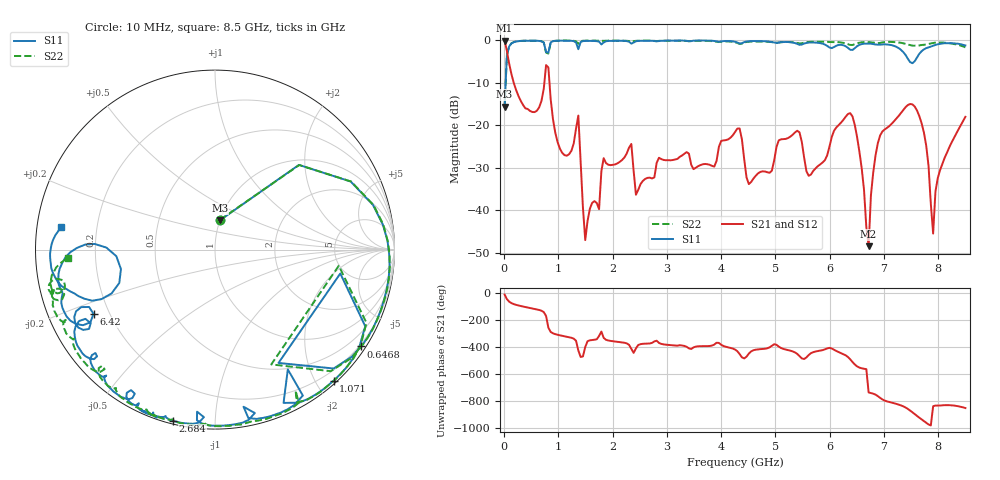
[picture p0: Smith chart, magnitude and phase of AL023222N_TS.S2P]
!AVX CORPORATION
!PN: AL023222N_TS
!DESCRIPTION: AIR CORE INDUCTOR, 222nH, 14 turns
!Agilent Technologies,E5071C,MY46102230,A.09.54
!Date: Mon Sep 03 16:46:35 2012
!Data & Calibration Information:
!Freq	S11:SOLT2(ON)	S21:SOLT2(ON)	S12:SOLT2(ON)	S22:SOLT2(ON)
# Hz S dB R 50
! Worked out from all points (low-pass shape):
!   201 points, 10 MHz to 8.5 GHz, reference 50 ohm
!   highest |S21| = -0.11 dB at 10 MHz (marker M1); lowest = -48.4 dB at 6.717 GHz (marker M2)
!   |S21| within 3 dB of the highest: start of sweep to 60.05 MHz
!   lowest |S11| = -15.6 dB at 10 MHz (marker M3), VSWR 1.40, Z = 50 + j16.8 ohm
!   |S11| at or under -10 dB: start of sweep to 29.75 MHz
!   |S22| runs from -15.5 to -0.1 dB; largest |S21 - S12| = 0.0023
!   S11 on the Smith chart (normalised r, x): 10 MHz: 1.00, +0.34; 646.8 MHz: 0.14, -3.32; 1.071 GHz: 0.05, -2.25; 2.684 GHz: 0.01, -0.78; 6.42 GHz: 0.14, -0.24; 8.5 GHz: 0.07, +0.07
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1e7  -15.61 80.4  -0.11 -10.2  -0.10 -10.2  -15.54 80.9
1.798e8  -0.49 8.5  -10.10 -81.1  -10.08 -81.1  -0.46 8.4
6.4675e8  -0.20 -33.5  -15.80 -124.4  -15.80 -124.4  -0.19 -34.1
8.1655e8  -2.97 -10.8  -6.44 103.8  -6.43 103.8  -3.15 -7.4
1.07125e9  -0.13 -47.8  -26.49 44.3  -26.48 44.2  -0.12 -47.1
1.3684e9  -2.14 -58.7  -17.74 -64.2  -17.73 -64.1  -0.87 -60.2
1.4533e9  -0.25 -62.9  -39.40 -108.3  -39.58 -108.7  -0.16 -63.9
2.34475e9  -0.83 -96.3  -24.40 -51.7  -24.40 -51.6  -0.35 -93.8
2.42965e9  -0.28 -95.4  -36.32 -48.9  -36.45 -49.9  -0.17 -95.0
2.68435e9  -0.15 -103.7  -32.31 -12.6  -32.38 -12.6  -0.12 -101.5
2.85415e9  -0.21 -107.0  -27.64 -8.4  -27.69 -8.4  -0.18 -104.6
4.255e9  -0.39 -121.1  -21.63 -57.3  -21.63 -57.3  -0.51 -133.4
4.5097e9  -0.28 -121.2  -33.82 -87.7  -33.85 -87.4  -0.39 -135.8
5.40115e9  -0.89 -139.4  -21.29 -89.5  -21.28 -89.5  -0.67 -154.8
5.6983e9  -0.57 -143.5  -30.71 -76.9  -30.83 -76.7  -0.40 -157.8
6.41995e9  -2.32 -152.1  -17.94 -149.9  -17.94 -149.9  -1.15 -163.5
6.7171e9  -0.82 -159.3  -48.41 -15.3  -48.10 -13.7  -0.48 -165.2
6.84445e9  -1.03 -163.4  -27.08 -31.5  -27.14 -31.8  -0.67 -165.9
7.09915e9  -1.09 -171.1  -20.18 -86.4  -20.18 -86.4  -0.42 -166.6
7.651e9  -3.22 -156.4  -17.86 157.7  -17.86 157.8  -1.25 -165.5
7.9057e9  -1.33 -165.2  -45.44 -117.2  -45.44 -120.6  -0.68 -165.2
8.5e9  -1.26 171.8  -18.03 -130.8  -18.03 -130.8  -1.70 -176.6
